FUNCTION_BLOCK FB_AxisPtp EXTENDS FB_AxisBase
VAR_INPUT
	Com								:	FB_Command;
END_VAR                 		
VAR_INPUT PERSISTENT    		
	Cfg								:	FB_Configure;
END_VAR
VAR_OUTPUT
	STO_Activate			AT%Q*	:	BOOL := TRUE;
END_VAR
VAR
	
END_VAR



M_Cyclic();

METHOD M_Cyclic : BOOL
VAR_INPUT
END_VAR
refAxis.ReadStatus();

M_Power(Com.bEnable,Com.bEnPos,Com.bEnNeg,COM.fOverride);

M_JogForward(Com.bJogFwd);

M_JogBackwards(Com.bJogBwd);

M_Reset(Com.bReset);

M_Stop(Com.bStop);

IF Com.nPtpMode = 1 THEN // 配合 hmi 使用
	M_MovRel(Com.bRun,Com.fPosition,Com.fVelocity);
ELSIF Com.nPtpMode = 2 THEN 
	M_MovAbs(com.bRun,com.fPosition,com.fVelocity);	
END_IF

M_GearIn(com.bGearIn,com.fRatio,com.nMasterAxisId);

M_GearOut(com.bGearOut);

// 备用
M_CamIn(com.bCamIn,com.nMasterAxisId,com.nCamTableID);
END_METHOD

END_FUNCTION_BLOCK
